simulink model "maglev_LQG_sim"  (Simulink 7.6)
settings: Solver=ode45  StartTime=0.0  StopTime=5  RelTol=1e-3
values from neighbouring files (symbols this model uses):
  Akf = A_maglev - Kkf * C_maglev    [design_KF_maglev.m]
  Bkf = [B_maglev Kkf]    [design_KF_maglev.m]
  C = C * 1e-5    [maglev_init.m]
  Ckf = eye(3)    [design_KF_maglev.m]
  Dkf = zeros(3,4)    [design_KF_maglev.m]
  g = 9.80665    [maglev_init.m]
  L1 = L1/10    [maglev_init.m]
  m = m/100    [maglev_init.m]
  R = input('Inserire le prime due cifre (esclusi zeri) del proprio numero di matricola:\n\n')    [maglev_init.m]
  x1_0 = 0.1    [maglev_init.m]
  x1_d = 0.05    [maglev_init.m]
  x2_0 = 0    [maglev_init.m]
  x2_d = 0    [maglev_init.m]
  x3_0 = 0.2    [maglev_init.m]
undefined symbols (not defined in the file or in its folder): K, mpert
libraries: simulink x2

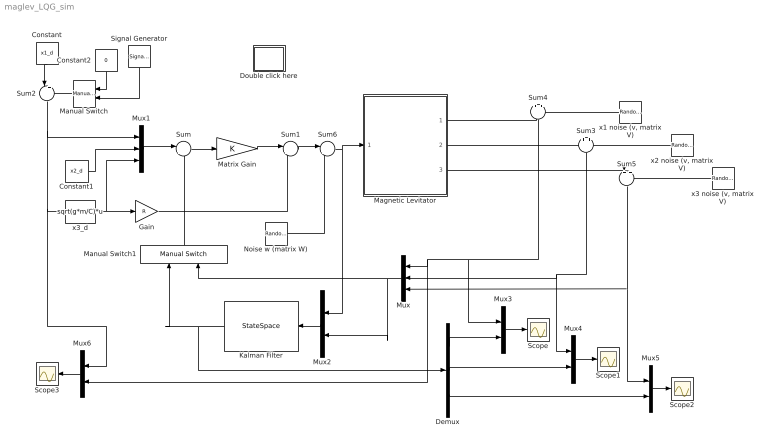
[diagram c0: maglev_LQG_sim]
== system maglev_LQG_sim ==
  Constant : Constant  Value=x1_d
  Constant1 : Constant  Value=x2_d
  Constant2 : Constant  Value=0
  Demux : Demux  Outputs=3
  Double click here : Subsystem
  Gain : Gain  Gain=R
  Kalman Filter : StateSpace  A=Akf  B=Bkf  C=Ckf  D=Dkf
  Magnetic Levitator : Subsystem  mask{m=m+mpert, R=R, L1=L1, C=C, g=g}
      mask prompts: m "ball's mass (m)"; R "Electromagnet's resistance (R)"; L1 "Electromagnet's inductance (L1)"; C "Magnetic force constant (C)"; g "Gravitational acceleration (g)"
  Manual Switch : simulink/Signal Routing/Manual Switch  SystemSampleTime=-1  sw=0  action=0  varsize=off
  Manual Switch1 : simulink/Signal Routing/Manual Switch  SystemSampleTime=-1  sw=0  action=0  varsize=off
  Matrix Gain : Gain  Gain=K  Multiplication=Matrix(K*u)
  Mux : Mux  Inputs=3
  Mux1 : Mux  Inputs=3
  Mux{2..6} (5 alike) : Mux  Inputs=2
  Noise w (matrix W) : RandomNumber  Seed=1  SampleTime=0
  Scope{,1..3} (4 alike) : Scope
  Signal Generator : SignalGenerator  WaveForm=square  Amplitude=x1_d*0.1  Frequency=0.5
  Sum : Sum  Inputs=|+-
  Sum1 : Sum  Inputs=|++
  Sum2 : Sum  Inputs=|++
  Sum3 : Sum  Inputs=+|+
  Sum4 : Sum  Inputs=+|+
  Sum5 : Sum  Inputs=+|+
  Sum6 : Sum  Inputs=|++
  "x1 noise (v, matrix V)" : RandomNumber  Variance=0.00001  Seed=2  SampleTime=0
  "x2 noise (v, matrix V)" : RandomNumber  Variance=0.00001  Seed=3  SampleTime=0
  "x3 noise (v, matrix V)" : RandomNumber  Variance=0.01  Seed=4  SampleTime=0
  x3_d : Fcn  Expr=sqrt(g*m/C)*u
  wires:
  x3_d/1 -> Mux1/3, Gain/1
  Constant1/1 -> Mux1/2
  Sum/1 -> Matrix Gain/1
  Mux/1 -> Manual Switch1/2, Mux2/2
  Mux1/1 -> Sum/1
  Matrix Gain/1 -> Sum1/1
  Gain/1 -> Sum1/2
  Constant/1 -> Sum2/1
  Constant2/1 -> Manual Switch/1
  Signal Generator/1 -> Manual Switch/2
  Manual Switch/1 -> Sum2/2
  Sum2/1 -> Mux1/1, x3_d/1, Mux6/1
  Magnetic Levitator/1(x1) -> Sum4/1
  Sum4/1 -> Mux3/1, Mux/1, Mux6/2
  Magnetic Levitator/2(x2) -> Sum3/1
  Sum3/1 -> Mux/2, Mux4/1
  Magnetic Levitator/3(x3) -> Sum5/1
  Sum5/1 -> Mux/3, Mux5/1
  Sum1/1 -> Sum6/1
  Sum6/1 -> Magnetic Levitator/1(u), Mux2/1
  Noise w (matrix W)/1 -> Sum6/2
  "x1 noise (v, matrix V)"/1 -> Sum4/2
  "x2 noise (v, matrix V)"/1 -> Sum3/2
  "x3 noise (v, matrix V)"/1 -> Sum5/2
  Mux2/1 -> Kalman Filter/1
  Kalman Filter/1 -> Demux/1, Manual Switch1/1
  Demux/1 -> Mux3/2
  Demux/2 -> Mux4/2
  Demux/3 -> Mux5/2
  Mux3/1 -> Scope/1
  Mux4/1 -> Scope1/1
  Mux5/1 -> Scope2/1
  Manual Switch1/1 -> Sum/2
  Mux6/1 -> Scope3/1

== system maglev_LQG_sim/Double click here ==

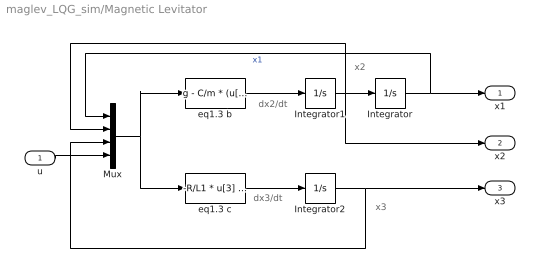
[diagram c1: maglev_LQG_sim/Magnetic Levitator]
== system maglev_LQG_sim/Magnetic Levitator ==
  note: x2
  note: x3
  note: dx2/dt
  note: dx3/dt
  u : Inport
  Integrator : Integrator  InitialCondition=x1_0
  Integrator1 : Integrator  InitialCondition=x2_0
  Integrator2 : Integrator  InitialCondition=x3_0
  Mux : Mux
  eq1.3 b : Fcn  Expr=g - C/m * (u[3] / u[1])^2
  eq1.3 c : Fcn  Expr=-R/L1 * u[3] + (2*C)/L1 * ( u[2] * u[3] / u[1]^2 ) + 1/L1 * u[4]
  x1 : Outport
  x2 : Outport  Port=2
  x3 : Outport  Port=3
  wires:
  eq1.3 b/1 -> Integrator1/1
  Integrator1/1 -> Integrator/1, Mux/2, x2/1
  eq1.3 c/1 -> Integrator2/1
  Mux/1 -> eq1.3 b/1, eq1.3 c/1
  Integrator/1 -> Mux/1, x1/1  "x1"
  Integrator2/1 -> Mux/3, x3/1
  u/1 -> Mux/4
